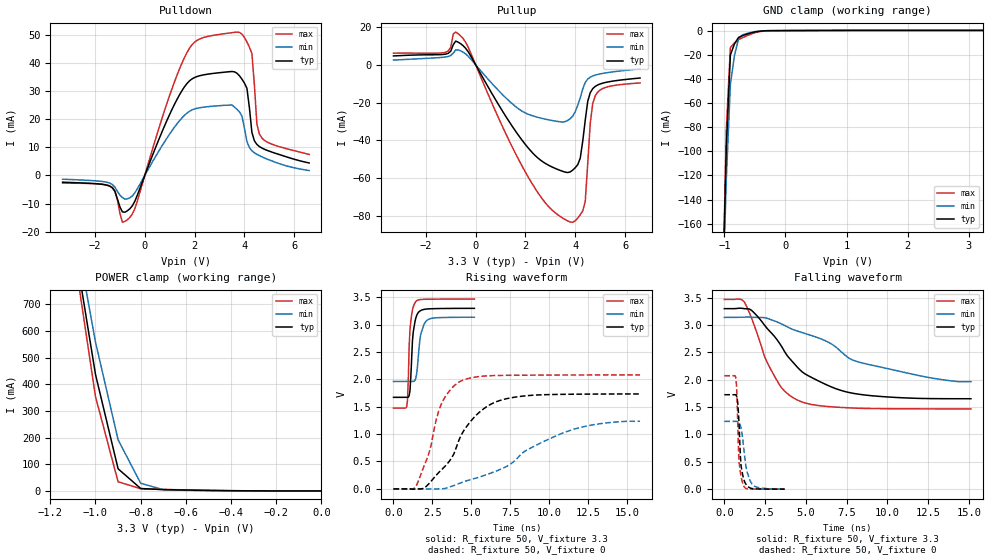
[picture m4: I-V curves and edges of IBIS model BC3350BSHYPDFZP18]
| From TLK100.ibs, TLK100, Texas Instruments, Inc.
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|   Model Cell BC3350BSHYPDFZP18
[Model]   BC3350BSHYPDFZP18
Model_type   I/O
Polarity   Non-Inverting
Enable   Active-Low
Vinl =  0.8V
Vinh =  2V
Cref =  15.0000pF
Rref =  100.0000M
Vref =  0V
Vmeas =  1.65
C_comp   1.737544p   1.689782p   1.779236p
[Model Spec]
Vinl   0.8V   0.8V   0.8V
Vinh   2V   2V   2V
[Temperature Range]   25   125   -40
[Voltage Range]   3.3   3.14   3.47
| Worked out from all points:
|   slope of the pulldown table from 0 to 0.495 V, typ, clamps not added: 44 ohm
|   slope of the pullup table from 0 to 0.495 V, typ, clamps not added: 42.8 ohm
|   GND clamp passes 1 mA (typ) near -0.49 V on its own axis
|   POWER clamp passes 1 mA (typ) near -0.40 V on its own axis
|   rising waveform, R_fixture 50, V_fixture 3.3: 20-80 % time 229ps typ, 310ps min, 186ps max; typ from 1.67 V to 3.3 V
|   rising waveform, R_fixture 50, V_fixture 0: 20-80 % time 2.39ns typ, 4.75ns min, 1.32ns max; typ from 0 V to 1.73 V
|   falling waveform, R_fixture 50, V_fixture 3.3: 20-80 % time 3.21ns typ, 5.73ns min, 1.74ns max; typ from 3.3 V to 1.65 V
|   falling waveform, R_fixture 50, V_fixture 0: 20-80 % time 202ps typ, 372ps min, 160ps max; typ from 1.73 V to 0.001 V
[POWER_clamp]
|   voltage   I(typ)   I(min)   I(max)
-3.3V     15.06A     13.65A     16.18A
-1.067V   785.8mA    871.3mA    732.8mA
-1.033V   611.7mA    715.2mA    543.5mA
-1V       437.6mA    559.1mA    354.2mA
-900mV    83.19mA    192.2mA    34.49mA
-800mV    9.176mA    28.76mA    8.234mA
-700mV    4.915mA    4.879mA    5.819mA
-400mV    992.9uA    605.1uA    994.2uA
-11.55fV  143uA      83.19uA    234.1uA
[Pulldown]
|   voltage   I(typ)   I(min)   I(max)
-3.3V     -2.42mA    -1.355mA   -2.742mA
-1.4V     -3.866mA   -2.765mA   -3.735mA
-900mV    -12.98mA   -7.875mA   -16.63mA
-700mV    -12.58mA   -8.35mA    -15.75mA
1.7V      32.7mA     22.18mA    43.75mA
3.6V      36.79mA    24.24mA    50.83mA
3.9V      34.2mA     21.08mA    50.21mA
4.1V      30.97mA    12.06mA    47.43mA
4.3V      15.29mA    8.758mA    43.35mA
4.5V      11.02mA    7.483mA    18.29mA
4.6V      10.26mA    7.017mA    14.72mA
6.6V      4.411mA    1.71mA     7.433mA
[Pullup]
|   voltage   I(typ)   I(min)   I(max)
-3.3V     4.71mA     2.514mA    6.161mA
-1.2V     5.694mA    4.171mA    6.671mA
-1V       7.232mA    4.973mA    9.382mA
-900mV    10.66mA    6.233mA    16.33mA
-600mV    11.14mA    7.389mA    15.31mA
2.2V      -45.34mA   -26.59mA   -61.37mA
3.8V      -56.6mA    -28.41mA   -83.18mA
4.2V      -49.34mA   -17.47mA   -79.29mA
4.4V      -29.22mA   -9.297mA   -72.12mA
4.6V      -14.75mA   -6.534mA   -31.03mA
4.8V      -11.42mA   -5.437mA   -16.4mA
6.6V      -6.969mA   -2.118mA   -9.572mA
[GND_clamp]
|   voltage   I(typ)   I(min)   I(max)
-3.3V     -17.31A    -15.65A    -18.51A
-1.033V   -232.2mA   -237.2mA   -236.9mA
-966.7mV  -97.23mA   -123.2mA   -82.64mA
-900mV    -20.26mA   -44.69mA   -13.99mA
-833.3mV  -11.04mA   -20.57mA   -10.21mA
-766.7mV  -5.656mA   -6.848mA   -7.493mA
-700mV    -4.119mA   -3.521mA   -5.837mA
-500mV    -1.109mA   -856.9uA   -1.751mA
-300mV    -91.67uA   -79.85uA   -139.7uA
3.233V    142.9uA    85.46uA    233.8uA
[Ramp]
| variable   typ   min   max
dV/dt_f  0.9938786/3.222725n   0.7649968/6.717107n   1.208123/1.739203n
dV/dt_r   1.04543/2.405617n   0.7664369/4.963119n   1.252704/1.327836n
R_load = 50
[Rising Waveform]
R_fixture = 50
V_fixture = 3.3
V_fixture_min = 3.14
V_fixture_max = 3.47
|   time   V(typ)   V(min)   V(max)
0s        1.671V     1.961V     1.476V
844ps     1.672V     1.962V     1.495V
896ps     1.672V     1.962V     1.612V
1.004ns   1.703V     1.962V     2.595V
1.056ns   1.789V     1.962V     2.904V
1.216ns   2.701V     1.961V     3.264V
1.428ns   3.116V     2.02V      3.419V
1.748ns   3.257V     2.823V     3.457V
2.116ns   3.283V     3.07V      3.462V
5.188ns   3.296V     3.135V     3.465V
[Rising Waveform]
R_fixture = 50
V_fixture = 0
V_fixture_min = 0
V_fixture_max = 0
|   time   V(typ)   V(min)   V(max)
0s        47.13uV    24.16uV    78.49uV
1.448ns   -2.152mV   -961uV     46.45mV
2.256ns   90.11mV    -451.5uV   634.9mV
3.064ns   345.1mV    989.8uV    1.547V
3.708ns   556.1mV    44.84mV    1.829V
4.352ns   988.6mV    114.6mV    1.973V
5.644ns   1.432V     228.5mV    2.056V
7.256ns   1.647V     411mV      2.073V
11.29ns   1.727V     1.065V     2.079V
15.8ns    1.733V     1.234V     2.081V
[Falling Waveform]
R_fixture = 50
V_fixture = 3.3
V_fixture_min = 3.14
V_fixture_max = 3.47
|   time   V(typ)   V(min)   V(max)
0s        3.297V     3.138V     3.465V
1.232ns   3.296V     3.141V     3.416V
1.692ns   3.26V      3.14V      3.105V
2.464ns   2.996V     3.133V     2.423V
3.084ns   2.786V     3.071V     2.059V
3.7ns     2.51V      2.99V      1.79V
4.624ns   2.183V     2.873V     1.609V
6.324ns   1.899V     2.693V     1.51V
8.02ns    1.745V     2.342V     1.48V
15.13ns   1.652V     1.964V     1.466V
[Falling Waveform]
R_fixture = 50
V_fixture = 0
V_fixture_min = 0
V_fixture_max = 0
|   time   V(typ)   V(min)   V(max)
0s        1.725V     1.238V     2.072V
716ps     1.718V     1.238V     2.013V
756ps     1.695V     1.239V     1.837V
832ps     1.545V     1.232V     1.095V
908ps     1.145V     1.21V      482.1mV
1.02ns    445.2mV    1.122V     242.1mV
1.208ns   164.6mV    701.6mV    47.51mV
1.4ns     61.58mV    308.4mV    6.944mV
1.74ns    10mV       80.5mV     1.953mV
3.704ns   940.7uV    3.177mV    128.8uV
